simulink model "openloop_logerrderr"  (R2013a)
settings: Solver=ode45  StartTime=0.0  StopTime=0.01  RelTol=1e-3
libraries: powerlib x16

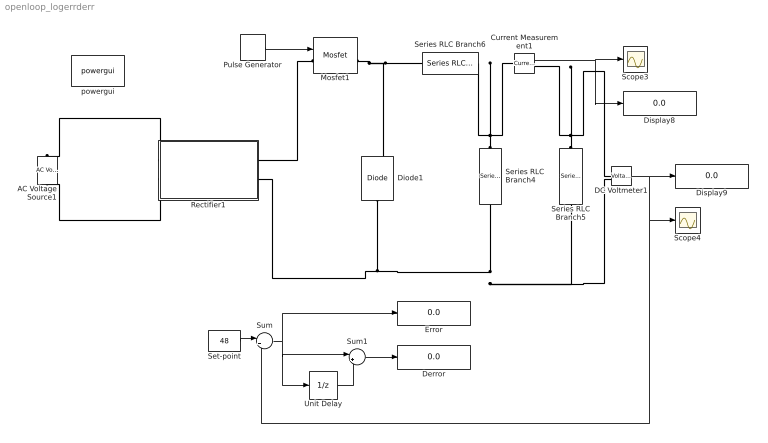
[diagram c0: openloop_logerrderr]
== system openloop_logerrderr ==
  AC Voltage Source1 : powerlib/Electrical Sources/AC Voltage Source  Amplitude=311.13  Phase=0  Frequency=50  SampleTime=0  Measurements=None
  Current Measurement1 : powerlib/Measurements/Current Measurement  PhasorSimulation=off  OutputType=Complex  PSBequivalent=0
  DC Voltmeter1 : powerlib/Measurements/Voltage Measurement  PhasorSimulation=off  OutputType=Complex  PSBequivalent=0
  Derror : Display
  Diode1 : powerlib/Power Electronics/Diode  Ron=0.001  Lon=0  Vf=0.8  IC=0  UseSnubber=off  Rs=500  Cs=250e-9  Measurements=on
  Display8 : Display
  Display9 : Display
  Error : Display
  Mosfet1 : powerlib/Power Electronics/Mosfet  Ron=0.1  Lon=0  Rd=0.01  Vfd=0  IC=0  Rs=1e5  Cs=inf  Measurements=on
  Pulse Generator : DiscretePulseGenerator  PulseType=Time based  Period=0.000025  PulseWidth=73
  Rectifier1 : Subsystem
  Scope3 : Scope
  Scope4 : Scope
  Series RLC Branch4 : powerlib/Elements/Series RLC Branch  LConnTagsString=__new0  RConnTagsString=__new0  BranchType=C  Resistance=1  Inductance=1e-3  SetiL0=off  InitialCurrent=0  Capacitance=1.35634e-05  Setx0=off  InitialVoltage=0  Measurements=None
  Series RLC Branch5 : powerlib/Elements/Series RLC Branch  LConnTagsString=__new0  RConnTagsString=__new0  BranchType=R  Resistance=9  Inductance=1e-3  SetiL0=off  InitialCurrent=0  Capacitance=1e-6  Setx0=off  InitialVoltage=0  Measurements=None
  Series RLC Branch6 : powerlib/Elements/Series RLC Branch  LConnTagsString=__new0  RConnTagsString=__new0  BranchType=L  Resistance=1  Inductance=0.0002304  SetiL0=off  InitialCurrent=0  Capacitance=1e-6  Setx0=off  InitialVoltage=0  Measurements=None
  Set-point : Constant  Value=48
  Sum : Sum  Inputs=|+-
  Sum1 : Sum  Inputs=|+-
  Unit Delay : UnitDelay  SampleTime=-1
  powergui : powerlib/powergui  Priority=1  SimulationMode=Continuous  SolverType=Tustin  SampleTime=2.5e-5  frequency=60  SPID=off  DisableSnubberDevices=off  DisableRonSwitches=off  DisableVfSwitches=off  SwTol=0  Interpol=off  DisplayEquations=off  frequencyindice=0  Pbase=100e6  ErrMax=1e-4  Iterations=50  UnitsV=kV  UnitsW=MW  FunctionMessages=off  echomessages=off  HookPort=off  EnableUseOfTLC=off  x0status=blocks  RestoreLinks=warning  ResistiveCurrentMeasurement=off  Frange=[0:2:500]  Ylog=off  Xlog=on  ShowGrid=off  save=off  variable=ZData  ZoomFFT=off  StartTime=0.0  cycles=1  DisplayStyle=1  fundamental=60  FreqAxis=off  MaxFrequency=1000  frequencyindicesteady=1  RmsSteady=2  display=off  Ts=0  methode=off
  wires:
  Current Measurement1/1 -> Scope3/1, Display8/1
  Pulse Generator/1 -> Mosfet1/1
  DC Voltmeter1/1 -> Sum/2, Scope4/1, Display9/1
  Unit Delay/1 -> Sum1/2
  Set-point/1 -> Sum/1
  Sum/1 -> Error/1, Unit Delay/1, Sum1/1
  Sum1/1 -> Derror/1
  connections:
  Diode1/LConn1 -- Series RLC Branch4/RConn1 -- Series RLC Branch5/RConn1 -- DC Voltmeter1/LConn2 -- Rectifier1/RConn2
  Mosfet1/RConn1 -- Series RLC Branch6/LConn1 -- Diode1/RConn1
  Series RLC Branch5/LConn1 -- Current Measurement1/RConn1 -- DC Voltmeter1/LConn1
  Series RLC Branch4/LConn1 -- Current Measurement1/LConn1 -- Series RLC Branch6/RConn1
  Rectifier1/LConn1 -- AC Voltage Source1/RConn1
  Rectifier1/LConn2 -- AC Voltage Source1/LConn1
  Mosfet1/LConn1 -- Rectifier1/RConn1

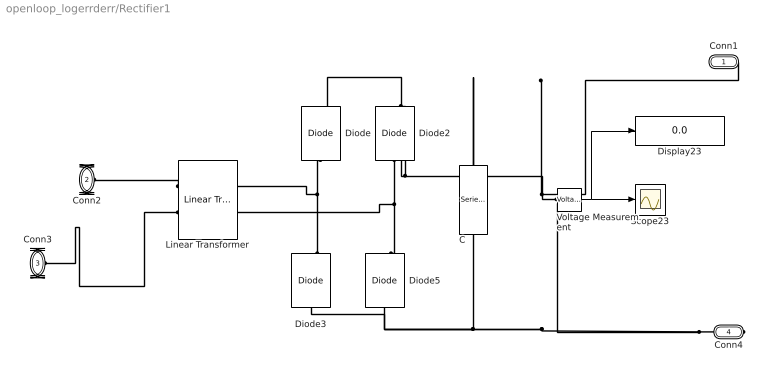
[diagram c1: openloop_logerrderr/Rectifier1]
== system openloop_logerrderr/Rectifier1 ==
  C : powerlib/Elements/Series RLC Branch  LConnTagsString=__new0  RConnTagsString=__new0  BranchType=C  Resistance=1  Inductance=1e-3  SetiL0=off  InitialCurrent=0  Capacitance=4859e-5  Setx0=off  InitialVoltage=0  Measurements=None
  Diode{,2..3,5} (4 alike) : powerlib/Power Electronics/Diode  Ron=0.001  Lon=0  Vf=0.8  IC=0  UseSnubber=off  Rs=500  Cs=250e-9  Measurements=on
  Display23 : Display
  Linear Transformer : powerlib/Elements/Linear Transformer  LConnTagsString=a|b  RConnTagsString=A|B  UNITS=pu  NominalPower=[ 1000 50 ]  winding1="[ 220  0  0 ]"  winding2="[ 48  0  0 ]"  ThreeWindings=off  winding3=[ 315e3 0.002 0.08 ]  RmLm=[ 500 500 ]  Measurements=None  DataType=off
  Scope23 : Scope
  Voltage Measurement : powerlib/Measurements/Voltage Measurement  PhasorSimulation=off  OutputType=Complex  PSBequivalent=0
  Conn1 : PMIOPort  Port=1  Side=Right
  Conn2 : PMIOPort  Port=2  Side=Left
  Conn3 : PMIOPort  Port=3  Side=Left
  Conn4 : PMIOPort  Port=4  Side=Right
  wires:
  Voltage Measurement/1 -> Display23/1, Scope23/1
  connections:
  Linear Transformer/LConn1 -- Conn2/RConn1
  Linear Transformer/LConn2 -- Conn3/RConn1
  Voltage Measurement/LConn1 -- C/LConn1 -- Diode/RConn1 -- Diode2/RConn1 -- Conn1/RConn1
  Diode2/LConn1 -- Diode5/RConn1 -- Linear Transformer/RConn2
  Diode3/RConn1 -- Linear Transformer/RConn1 -- Diode/LConn1
  Conn4/RConn1 -- Voltage Measurement/LConn2 -- Diode3/LConn1 -- Diode5/LConn1 -- C/RConn1
